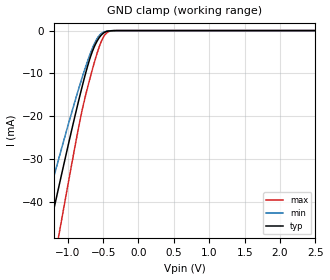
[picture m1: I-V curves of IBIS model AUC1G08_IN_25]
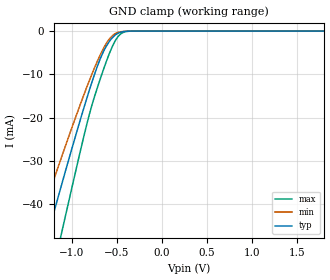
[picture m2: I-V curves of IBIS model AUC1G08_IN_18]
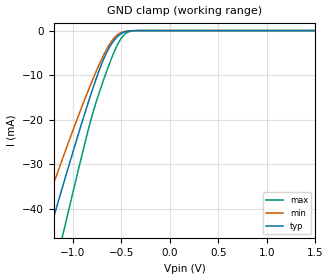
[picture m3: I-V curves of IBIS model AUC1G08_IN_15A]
| TEXAS INSTRUMENTS INCORPORATED
| Standard Linear and Logic Group
| IBIS Model of SN74AUC1G08
| Single 2-Input Positive-AND Gate
| This file contains package information for the following:
|  SOT 5-pin (DCK) package as [Component] AUC1G08_DCK
|  SOT 5-pin (DBV) package as [Component] AUC1G08_DBV
|  NanoFree WCSP 5-pin (YZP) package as [Component] AUC1G08_YZP
| This device can be powered at the following Vccs:
|  2.5 volt Vcc
|  1.8 volt Vcc
|  1.5 volt Vcc
|  1.2 volt Vcc
|  0.8 volt Vcc
| This file provides unique models under the [Model Selector] for each Vcc.
| For operation at a specific Vcc, select the appropriate model after each
| [Model Selector] keyword.
[IBIS Ver]   3.2
[Comment char]  |_char
[File Name]   sn74auc1g08.ibs
[File Rev]   1.4 | x_die
[Date]   April 10, 2006
[Source]   Data created from TI-SPICE simulations at TI-SLL.
[Notes]   The following is an IBIS list for the SN74AUC1G08.
   Please contact sllibis@ti.com with questions and
   comments concerning SLL IBIS models.
   - FILE REV HISTORY
   - 1.4 updated IBIS file on 04/17/08
   - Non-monotonic data in pullup and pulldown due to feedback
   circuit.
   - Power clamp data deleted as there is no power-clamp diode.
   - End point warning due to AC and DC mismatch.
[Disclaimer] Property of Texas Instruments Incorporated.  Unauthorized
   reproduction and/or distribution is strictly prohibited.
   This product is protected under copyright law.
   Created  2006, (C) Copyright  2006, Texas Instruments
   Incorporated, All Rights Reserved
   UNLESS THERE IS A SIGNED, WRITTEN AGREEMENT TO THE
   CONTRARY, TEXAS INSTRUMENTS (TI) IS PROVIDING THE IBIS
   MODELS  AND WITHOUT ANY WARRANTY, EXPRESSED OR
   IMPLIED.  TI assumes no liability for:
   1) the accuracy of the IBIS models provided to your
   company;
   2) the proper functioning of these IBIS Models in your
   design or for any resulting applications; or
   3) infringement of patents, copyrights or intellectual
   property rights resulting from your use of these IBIS
   models.
   TI provides IBIS Models as a service to our customers.
   You and your company shall not distribute, sell or give
   these models to anyone else without prior written
   permission from TI.
   TI reserves the right to make changes to our products or
   to discontinue any semiconductor product or service
   without notice, and advises our customers to obtain the
   latest version of relevant information to verify, before
   placing orders, that the information being relied on is
   current.
   Please be aware that your receipt and use of the IBIS
   information provided shall serve as acceptance of these
   terms and conditions.  If you do not accept these terms,
   you should return or destroy the IBIS models and any
   other accompanying information immediately.
| Component SN74AUC1G08_DCK 5-PIN SOT
[Component]   SN74AUC1G08_DCK
[Manufacturer]   Texas Instruments, Inc.
[Package]
|   typ   min   max
R_pkg   2.000e-02   1.700e-02   2.500e-02
L_pkg   9.980e-10   8.810e-10   1.069e-09
C_pkg   1.460e-13   1.180e-13   2.050e-13
[Pin]   signal_name   model_name   R_pin   L_pin   C_pin
1   A   AUC1G08_IN   1.900e-02   1.069e-09   1.620e-13
2   B   AUC1G08_IN   1.800e-02   8.810e-10   1.210e-13
3   GND   GND   1.700e-02   1.031e-09   2.050e-13
4   Y   AUC1G08_OUT   2.000e-02   9.600e-10   1.240e-13
5   VCC   POWER   2.500e-02   1.049e-09   1.180e-13
| Component AUC1G08_DBV 5-pin SOT
[Component]   AUC1G08_DBV
[Manufacturer]   Texas Instruments, Inc.
[Package]
|   typ   min   max
R_pkg   2.500e-02   2.100e-02   2.900e-02
L_pkg   1.529e-09   1.312e-09   1.906e-09
C_pkg   1.560e-13   1.100e-13   2.400e-13
[Pin]   signal_name   model_name   R_pin   L_pin   C_pin
1   A   AUC1G08_IN   2.100e-02   1.511e-09   1.440e-13
2   B   AUC1G08_IN   2.300e-02   1.312e-09   1.380e-13
3   GND   GND   2.900e-02   1.906e-09   2.400e-13
4   Y   AUC1G08_OUT   2.600e-02   1.541e-09   1.500e-13
5   VCC   POWER   2.500e-02   1.374e-09   1.100e-13
| Component AUC1G08_YZP 5-pin NanoStar WCSP
[Component]   AUC1G08_YZP
[Manufacturer]   Texas Instruments, Inc.
[Package]
|   typ   min   max
R_pkg   0.001   0.001   0.001
L_pkg   0.021nH   0.021nH   0.021nH
C_pkg   0.046pF   0.045pF   0.047pF
[Pin]   signal_name   model_name   R_pin   L_pin   C_pin
1   A   AUC1G08_IN   0.001   0.021nH   0.046pF
2   B   AUC1G08_IN   0.001   0.021nH   0.047pF
3   GND   GND   0.001   0.021nH   0.046pF
4   Y   AUC1G08_OUT   0.001   0.021nH   0.045pF
5   VCC   POWER   0.001   0.021nH   0.045pF
| Model AUC1G08_IN
[Model Selector]   AUC1G08_IN
AUC1G08_IN_25   2.5 volt Vcc
AUC1G08_IN_18   1.8 volt Vcc
AUC1G08_IN_15A   1.5 volt Vcc
AUC1G08_IN_12   1.2 volt Vcc
AUC1G08_IN_08   0.8 volt Vcc
| Model AUC1G08_OUT
[Model Selector]   AUC1G08_OUT
AUC1G08_OUT_25   2.5 volt Vcc
AUC1G08_OUT_18   1.8 volt Vcc
AUC1G08_OUT_15A   1.5 volt Vcc
AUC1G08_OUT_12   1.2 volt Vcc
AUC1G08_OUT_08   0.8 volt Vcc
| Models and submodels in the file (10): AUC1G08_IN_25 (Input), AUC1G08_IN_18 (Input), AUC1G08_IN_15A (Input), AUC1G08_IN_12 (Input), AUC1G08_IN_08 (Input), AUC1G08_OUT_25 (Output), AUC1G08_OUT_18 (Output), AUC1G08_OUT_15A (Output), AUC1G08_OUT_12 (Output), AUC1G08_OUT_08 (Output)
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[Model]   AUC1G08_IN_25
Model_type  Input
Vinl=0.7
Vinh=1.7
| variable   typ   min   max
C_comp   2.22pF   1.83pF   2.72pF
[Temperature Range]   40   100   -40
| Ambient temperature   25   85   -40
[Voltage range]   2.5   2.3   2.7
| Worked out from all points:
|   GND clamp passes 1 mA (typ) near -0.52 V on its own axis
[GND Clamp]
| AUC1G08_IN_25
|   Voltage   I(typ)   I(min)   I(max)
-3.6V     -228.2mA   -191.9mA   -274.5mA
-1.435V   -59.77mA   -48.97mA   -76.34mA
-1.385V   -55.96mA   -45.83mA   -71.72mA
-1.285V   -48.38mA   -39.6mA    -62.49mA
-1.24V    -44.99mA   -36.82mA   -58.34mA
-1.115V   -35.66mA   -29.22mA   -46.83mA
-835mV    -15.66mA   -13.06mA   -21.7mA
-715mV    -8.096mA   -6.92mA    -13.03mA
-610mV    -3.273mA   -2.635mA   -6.669mA
-495mV    -599.4uA   -381.2uA   -1.523mA
-340mV    -10.37uA   -9.312uA   -15.22uA
2.5V      453pA      1.243nA    77.67pA
[Model]   AUC1G08_IN_18
Model_type  Input
Vinl=0.5775
Vinh=1.2675
| variable   typ   min   max
C_comp   2.29pF   1.92pF   2.73pF
[Temperature Range]   40   100   -40
| Ambient temperature   25   85   -40
[Voltage range]   1.8   1.65   1.95
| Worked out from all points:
|   GND clamp passes 1 mA (typ) near -0.52 V on its own axis
[GND Clamp]
| AUC1G08_IN_18
|   Voltage   I(typ)   I(min)   I(max)
-3.6V     -228.2mA   -191.9mA   -274.5mA
-1.425V   -59.01mA   -48.34mA   -75.41mA
-1.375V   -55.2mA    -45.2mA    -70.8mA
-1.28V    -48mA      -39.29mA   -62.03mA
-1.235V   -44.61mA   -36.51mA   -57.88mA
-1.12V    -36.03mA   -29.52mA   -47.29mA
-1.085V   -33.45mA   -27.42mA   -44.08mA
-815mV    -14.32mA   -11.98mA   -20.07mA
-695mV    -6.998mA   -5.997mA   -11.76mA
-550mV    -1.556mA   -1.089mA   -3.594mA
-450mV    -219.9uA   -142.2uA   -558uA
1.8V      305pA      941.3pA    47.06pA
[Model]   AUC1G08_IN_15A
Model_type  Input
Vinl=0.49
Vinh=1.04
| variable   typ   min   max
C_comp   2.32pF   1.97pF   2.73pF
[Temperature Range]   40   100   -40
| Ambient temperature   25   85   -40
[Voltage range]   1.5   1.4   1.6
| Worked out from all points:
|   GND clamp passes 1 mA (typ) near -0.52 V on its own axis
[GND Clamp]
| AUC1G08_IN_15A
|   Voltage   I(typ)   I(min)   I(max)
-3.6V     -228.2mA   -191.9mA   -274.5mA
-1.365V   -54.44mA   -44.57mA   -69.87mA
-1.23V    -44.24mA   -36.21mA   -57.42mA
-1.11V    -35.29mA   -28.91mA   -46.37mA
-1.065V   -31.98mA   -26.22mA   -42.24mA
-815mV    -14.32mA   -11.98mA   -20.07mA
-700mV    -7.266mA   -6.224mA   -12.08mA
-580mV    -2.329mA   -1.757mA   -5.052mA
-515mV    -878.5uA   -571.2uA   -2.17mA
-460mV    -279.1uA   -178.4uA   -715.8uA
-315mV    -4.754uA   -4.764uA   -5.622uA
1.5V      253.5pA    827.4pA    37.13pA
